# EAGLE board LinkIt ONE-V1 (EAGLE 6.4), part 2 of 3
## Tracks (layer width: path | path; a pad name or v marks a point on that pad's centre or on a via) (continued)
GND  (via drill 0.1 pad 0.25 layers 1-2, 0.1 pad 0.25 layers 15-16, 0.2 pad 0.41 (continued)
  Bottom 0.102: U7.F4 U7.D4 | U7.F6 U7.F7 | U7.F7 U7.G7 | U7.H6 U7.H7 U7.H8 U7.J8 | U7.H6 U7.G6 U7.F6 | U7.J6 U7.J5 | U7.J6 U7.H6 | U7.J6 U7.K6 | U7.J6 U7.J7 | U7.J7 35.34,76.69 35.38,76.73 U7.J8 | U7.J7 35.38,76.33 | U7.F6 36.6,75.93 36.6,75.92 36.55,75.92 | U7.N8 U7.N9 | U7.E2 36.94,74.58 v36.96,74.6 | U3.PAD 36.2,83.34 36.2,82.98 37.47,81.71 37.47,81 36.96,80.49 v36.7,80.49 36.5,80.49 36.14,80.85 34.98,80.85 | 34.98,80.85 v31.42,80.85 | 62.89,97.59 X2.2 62.98,97.36 | X2.1 62.98,97.36 | U7.L2 U7.L1 | 32.73,73.73 32.87,73.87 33.33,74.33 U7.P2 v33.35,74.35 | 62.98,97.36 C38.2 | C38.2 | v34.98,80.8 34.98,80.85 | U7.G2 36.16,74.33 36.45,74.04 36.45,73.25 35.38,72.19 v35.38,72.06 | U7.F7 v36.55,76.33 | C131.2 C129.2 | U7.K1 | v43.16,79.53 43.21,79.58 43.16,79.63 | 43.54,80.01 43.69,80.01
  Bottom 0.127: 34.55,74.33 34.87,74.65 34.87,75.06 v35.33,75.51 | v31.85,75.21 32.74,75.21 33,75.46 33,76.07 | v36.6,72.06 36.6,72.62 37.01,73.03 37.01,73.63
  Bottom 0.132: v38.05,69.29 38.94,68.4 | v41.68,75.97 41.45,75.97 arc45 41.11,75.83 41.02,75.74 arc-45 40.72,75.62 39.52,75.62
  Bottom 0.152: U2.14 56.54,93.32 56.71,93.15 59.56,93.15 C37.2 | 53.74,82.07 U1.E1 53.51,82.3 52.02,82.3 v51.89,82.42 | U1.K1 53.76,85.16 v53.37,85.55 | v43.21,75.21 43.16,75.21 43.05,75.31 | 43.05,75.31 41.52,75.31 arc45 41.27,75.21 41.02,74.95 v41.02,74.85 | U2.29 54.14,96.17 54.65,96.69 U2.PAD | 43.05,75.31 45.47,75.31 47.45,73.33 50.22,73.33 | U7.D4 U7.C5 U7.B6 | v40.56,70.08 40.56,69.93 40.97,69.52 47.37,69.52 50.27,72.41 v51.33,72.41 | v38,72.72 38,70.46 41.04,67.41 arc45 41.48,67.23 48.29,67.23 49.25,68.2 52.65,68.2 | 51.03,73.33 v51.33,73.33 v52.86,73.33 v54.28,73.33 v55.8,73.33 | v6.43,94.36 6.43,95.07 J4.C5 | v16.51,88.9 16.51,87.83 15.39,86.71 15.39,74.76 19.04,71.1 27.92,71.1 29.9,73.08 | 25.42,72.62 26.29,71.75 27.63,71.75 29.62,73.74 32.74,73.74 32.87,73.87 | 31.57,72.52 31.32,72.77 30.43,72.77 28.65,70.99 28.65,70.41 28.57,70.33 | v55.12,64.03 55.09,64.01 55.09,62.61 54.74,62.25 54.62,62.25 R56.2 53.98,61.59 53.21,61.59 52.07,62.74 52.07,63.22 v52.17,63.32 52.15,63.32 52.2,63.27 52.86,63.27 53.54,63.96 C130.2 | 28.88,76.48 28.88,76.38 29.39,75.87 30.45,75.87 30.99,75.34 v31.47,75.34 | 53.98,78.26 53.98,79.02 54.38,79.43 54.53,79.43 54.74,79.63 | X3.4 44.55,74.62 v44.81,74.88 | 43.16,79.63 43.54,80.01 | 43.16,79.58 v43.16,79.53 v43.16,78.97 42.69,78.5 C113.2 | 45.29,79.98 v45.29,80.03 | 50.93,64.4 R75.1 | v40.46,69.11 40.46,68.78 41.15,68.1 v41.38,68.1 | v38.68,72.72 38.68,70.79 39.5,69.98 | v39.29,72.67 39.29,71.45 39.75,70.99 | v37.36,72.47 v37.36,71.4 | v37.36,71.4 37.34,71.37 | v37.36,71.4 37.36,71.37 37.39,71.35 37.39,70.03 37.44,69.98 | 58.55,81.3 58.8,81.3 59.46,80.64 v60.12,80.64
  Bottom 0.152: R6.2 49.82,82.21 | U7.M3 U7.L2 34.55,74.33 | v35.38,72.06 35.38,70.74 34.93,70.28 34.87,70.28 34.72,70.13
  Bottom 0.203: 45.8,77.44 C110.2 45.61,77.48 45.29,77.8 45.29,79.98 45.03,80.24 L15.1 | 59.13,75.26 69.84,75.26 v70.07,75.49 | v72.16,77.34 72.19,77.32 72.19,75.97 70.62,74.41 47.67,74.41 46.1,75.97 v45.54,75.97 v44.73,75.97 | U2.8 55.16,96.17 54.65,96.69 | U2.46 56.14,98.56 55.63,98.04 | 55.26,82.1 U1.F4 U1.F6 U1.F7 | 15.47,97.81 JTAG.2 | v44.73,75.97 44.7,75.95 | v44.73,75.97 44.09,75.97 | 44.09,75.97 44.07,75.95 | 44.09,75.97 v43.21,75.97 | v43.21,75.97 43.18,75.95 | v43.21,75.97 42.44,75.97 | 42.44,75.97 42.42,75.95 | 42.44,75.97 v41.68,75.97 41.66,75.95 | U7.J5 v35.33,75.53 | v35.33,75.53 U7.J8 U7.H8 | U7.H8 | U7.H8 U7.H6 | 46.1,77.24 48.03,75.31 54.72,75.31 C15.2 | v35.33,75.53 v35.33,75.52 v35.33,75.51 | U1.E1 53.76,82.13 53.57,82.32 51.99,82.32 v51.89,82.42 | U1.D4 55.26,82.1 | 55.26,82.1 v55.27,82.12 | 58.95,72.41 58.95,72.31 | 58.95,71.65 v58.95,71.6 | U1.C5 56.13,80.67 v56.66,80.67 | U1.B8 57.26,80.92 v57.23,80.95 | U1.D9 57.29,81.55 v57.28,81.56 | 58.6,84.4 58.6,84.45 58.6,84.58 v59.05,85.04 | 50.85,80.55 v50.81,80.58 | v10.52,59.89 10.59,59.89 10.74,59.74 12.75,59.74 12.93,59.92 12.93,61.82 12.95,61.85
  Bottom 0.254: 40.72,76.33 v40.74,76.3 40.16,76.3 v39.8,76.66 | 36.54,75.77 U7.F6 U7.H6 34.93,75.93 34.93,75.92 | 36.54,75.77 36.54,75.14 36.55,75.13 U7.D4 | 35.38,76.33 U7.H7 | U7.G7 U7.H7 | U7.G7 v36.55,76.33 36.55,75.77 36.54,75.77 | U7.G7 U7.G6 | U7.H7 U7.H6 | U7.H7 U7.H8 | U7.D4 U7.D2 U7.E2 36.96,74.33 v36.96,74.6 | U7.A2 38.65,74.33 v38.99,73.99 | 39.73,76.73 v39.8,76.66 | U7.A8 38.68,76.73 38.79,76.83 39.62,76.83 v39.8,76.66 | v58.61,79.9 58.41,79.9 U1.A10 U1.B9 57.73,80.55 | 57.75,81.53 U1.D9 U1.D7 U1.D6 U1.C6 56.26,81.03 | U1.B1 53.42,80.55 53.32,80.44 50.95,80.44 v50.81,80.58 | U7.L2 v34.54,73.94 v34.56,73.93 U7.K1
  Bottom 0.305: J4.P5 18.79,92.42 18.67,92.3 18.67,87.07 17.68,86.08 17.68,81.24 18.66,80.26 20.83,80.26 23.97,77.12 28.24,77.12 28.88,76.48 28.9,76.45 C76.2 | C60.2 25.42,72.62 24.81,72.01 19.13,72.01 16.38,74.76 16.38,86.61 17.6,87.83 17.6,89.43 17.3,89.74 16.64,89.74 | C38.2 60.08,97.19 60.33,96.95 60.33,96.3 C39.2 | 16.64,89.74 15.72,89.74 15.37,89.38 15.37,87.81 14.4,86.84 14.4,74.78 18.85,70.33 28.57,70.33 28.8,70.33 30.37,68.77 34.38,68.77 34.72,69.11 34.72,70.02 C92.2 | 16.64,89.74 v16.66,89.76 | 57.73,80.55 57.73,80.54 | U1.C9 U1.B9 | U1.B8 | v77.52,99.95 77.57,99.9 GPS.GND1 80.85,99.9 81.61,100.66 GPS.GND3 81.61,101.93 80.85,102.69 GPS.GND2 78.31,102.69 v78.18,102.56 | WI-FI/BT.GND1 83.9,81.91 84.2,82.22 WI-FI/BT.GND3 84.2,84 83.49,84.71 WI-FI/BT.GND2 80.92,84.71 v80.8,84.58 | WI-FI/BT.GND1 82.57,81.91 82.52,81.97 | 82.52,81.97 82.63,81.97 WI-FI/BT.GND1 | 82.52,81.97 80.87,81.97 v80.8,82.04 | v80.77,66.8 80.9,66.93 GSM.GND2 83.59,66.93 84.2,66.32 GSM.GND3 84.2,64.8 83.54,64.13 GSM.GND1 80.9,64.13 v80.64,64.39 | v55.75,74.35 57.07,74.35 57.12,74.3 | X3.2 41.94,72.59 v42.24,72.29 | v50.81,80.58 50.41,80.58 49.86,80.03 49.86,79.9 C6.2
  Bottom 0.406: C26.2 C39.2 | C38.2 60.08,97.88 v60.07,97.89 | C42.2 55.55,102.79 | C5.2 v33.02,95.4 33.05,95.38 | 53.98,78.26 53.98,77.65 53.57,77.24 v53.57,76.28 | C66.2 23.47,86.61 25.02,85.06 | C6.2 49.4,79.86 v49.39,79.87 | U11.35 65.02,81.41 | U11.35 66.17,80.14 | U11.35 66.17,82.55 | 67.31,81.41 U11.35 | v13.18,76.53 13.18,74.45 18.54,69.09 28.47,69.09 29.8,67.76 35.12,67.76 36.07,68.71 36.07,69.96 R104.2
  Bottom 0.457: 50.22,73.33 50.76,73.33 | 55.83,73.33 51.03,73.33 47.07,73.33 46.86,73.53
  Bottom 0.508: 55.83,73.33 56.01,73.15 58.12,73.15 58.95,72.31 58.95,71.65
  other vias: 34.14,77.93 36.54,75.13 36.54,75.53 35.34,76.33 35.73,75.93 35.74,76.56 33.74,77.13 38.68,71.86 37.41,69.98 38.73,70.82 39.5,73.48 40.16,71.96 40.92,71.3 40.51,73.89 42.34,71.63 41.02,73.89 40.67,75.59 42.39,75.97 44.02,75.97 45.49,75.16 42.8,75.16 43.61,75.16 44.37,75.16 45.14,75.16 45.14,76.17 44.37,76.17 43.61,76.23 42.8,76.23 31.17,81.76 41.22,76.83 58.29,101.73 61.09,101.73 61.98,101.73 61.09,99.82 61.98,99.82 59.82,99.82 62.99,99.82 62.99,103 64.26,103 65.53,103 66.8,103 68.07,103 68.96,98.81 68.96,99.82 68.07,100.97 69.34,103 70.61,103 71.88,103 73.15,103 70.61,100.46 71.88,100.46 73.15,100.46 75.06,103 75.06,100.46 76.17,100.46 52.93,88.44 78.13,84.58 78.13,83.31 78.26,82.04 79.53,82.04 78.26,80.77 79.65,81.15 77.9,77.72 75.59,77.6 75.46,79.88 79.4,79.12 59.99,78.41 60.63,77.65 61.43,77.09 62.76,76.96 64.16,76.96 65.11,76.96 65.18,79.38 63.59,79.38 62.32,79.38 61.37,79.18 60.76,80.09 67.74,76.81 70.05,79.76 68.35,79.76 71.2,79.76 72.39,79.76 72.92,76.96 70.03,76.23 51.31,75.31 57.84,75.34 45.29,77.9 45.29,78.97 44.53,80.9 44.58,70.84 42.34,70.94 52.86,72.42 54.28,72.42 55.17,72.42 51.33,71.5 52.86,71.5 54.28,71.5 51.36,69.52 52.71,69.32 51.89,66.88 78.84,78.1 61.37,73.91 42.6,62.76 45.21,64.97 46.28,64.97 47.29,64.97 49.28,62.94 39.93,67.36 39.52,69.95 39.29,67.89 40.41,67.03 59.82,68.07 61.72,68.07 61.72,69.98 62.99,69.98 64.26,69.98 65.53,69.98 66.8,69.98 68.07,69.34 66.8,68.07 65.53,68.07 64.26,68.07 62.99,68.07 70.48,64.9 69.6,67.94 68.07,66.8 71.25,66.55 69.34,65.53 73.02,66.29 71.88,64.9 74.55,66.17 75.69,66.8 75.56,64.9 73.79,64.9 77.6,66.8 77.6,64.9 79.38,64.9 26.59,77.7 24.71,80.54 25.78,79.43 22.58,80.7 23.9,81.36 20.9,82.17 14.35,83.77 14.4,81.86 16.38,81.81 16.38,83.77 17.65,81.81 7.65,81.2 9.22,81.15 10.54,81.15 16.46,77.72 25.25,103 21.74,102.21 54.74,96.65 55.73,89.18 56.03,90.09 59.69,89.13 55.55,103 54.28,102.97 56.92,103 50.62,102.69 52.83,98.55 54.74,98.55 56.64,98.55 52.83,96.65 56.64,96.65 56.64,94.74 54.74,94.74 52.83,94.74 55.42,85.5 19.66,94.18 19.71,92.91 13.72,97.08 6.81,98.7 28.37,94.87 29.34,92.63 11.1,83.03 24.61,75.26 24.66,74.55 24.66,73.74 36.6,75.21 38.89,73.63 38.89,73.08 33.81,74.09 38.13,82.42 38.58,82.42 36.75,82.47 35.59,82.47 34.26,82.47 50.04,62.92 42.34,68.22 40.21,72.92 40.82,72.31 12.6,91.85 20.75,80.34 18.62,80.29 17.3,79.76 54.64,69.95 56.03,69.95 57.56,69.95 56.03,68.68 57.56,68.68 54.64,68.68 54.64,67.41 55.91,67.41 57.56,67.41 53.85,98.55 55.75,98.55 53.72,96.65 55.75,96.65 53.72,94.74 55.75,94.74 52.83,95.63 52.83,97.66 53.85,97.66 54.74,97.66 55.75,97.66 56.64,97.66 56.64,95.63 55.75,95.63 54.74,95.63 53.72,95.63 44.45,74.63 44.02,75.26 44.73,75.26 42.42,75.26 41.66,75.29 39.27,71.86 39.55,71.15 40.01,70.69 36.96,69.42 37.47,69.42 38.96,69.44 38,71.86 38,70.84 38.38,70.03 39.85,68.55 52.55,68.2 52.1,71.5 57.84,74.32 51.33,74.3 52.86,74.3 54.23,74.35 52.86,75.31 57.12,73.15 36.52,75.92 37.01,74.88 37.36,74.42 37.8,73.99 31.17,82.83 31.17,84 30.86,80.24 29.95,80.99 29.79,84.25 40.69,78.33 33.12,74.04 15.37,83.77 15.37,81.86 15.37,80.31 16.38,80.31 14.4,80.31 29.84,73.08 21.03,92.86 21.69,93.22 22,94.34 20.57,93.62 49.05,95.2 49,96.22 44.58,69.52 44.58,68.38 46.46,71.81 46.46,70.84 46.46,69.52 46.41,68.38 27.41,77.72 27.18,80.44 25.2,80.01 44.58,66.47 37.29,73.43 37.85,73.43 38.46,73.43 38.46,73.99 13.18,80.37 13.18,77.7 17.4,77.7 36.65,72.62 35.43,71.45 2.03,92.89 2.03,90.35 5.33,92.89 5.21,90.22 2.03,87.81 5.21,87.81 15.37,58.55 16.64,58.55 58.04,62.79 60.45,62.36 62.99,62.36 62.99,64.26 62.99,66.17 59.82,66.17 70.61,61.72 73.79,61.72 75.82,61.72 78.23,61.72 81.41,57.28 81.41,61.72 61.72,70.99 65.91,73.91 70.61,57.28 70.1,73.91 69.34,70.61 76.96,73.91 76.96,70.36 82.04,73.79 82.04,70.61 69.98,84.58 75.95,82.04 69.98,92.2 75.69,92.2 82.04,92.2 68.96,97.92 80.14,97.92 55.37,88.39 57.28,88.39 0.89,78.1 50.72,85.6 12.19,98.6 12.19,101.14 10.29,101.14 5.21,101.14 10.29,107.37 28.52,73.36 71.88,78.36 66.67,78.1 30.58,75.21 30.58,73.94 32.77,71.81 32.61,73.66 32.61,73.03 31.8,73.08 35,72.69 35.56,72.69 48.64,91.08 24.99,85.09 22.35,90.32 31.22,77.11 41.96,78.45 41.2,78.33 41.2,77.88 40.69,77.88 35.71,78.08 34.7,78.03 36.88,76.17 36.6,75.82 40.94,67.46 48.69,75.82 48.74,72.44 48.74,69.01 48.74,69.65 25.29,73.72 42.47,66.45 30.61,73.48 31.32,73.48 30.61,72.57 31.32,72.57 30.58,73.05 31.45,74.04 62.76,73.91 64.03,73.91 58.7,75.31 58.7,74.3 68.22,73.91 23.13,79.77 36.17,72.69 32.74,72.42 42.82,80.21 61.77,87.76 32.49,103.38 38.84,103.25 42.52,100.33 43.03,96.52 46.71,102.74 46.71,100.46 46.71,98.04 49,93.47 50.77,90.55 51.41,91.19 38.33,90.3 19.81,58.55 19.81,57.91 77.01,77.72 77.01,78.99 78.03,79.5 75.49,78.87 75.95,83.31 76.07,85.85 33.07,71.02 34.29,71.02 35.51,71.02 31.8,71.02 59.11,79.43 48.4,76.52 59.82,73.91 59.82,71.88 61.72,71.88 70.03,77.5 59.66,85.55 64.48,79.38 30.2,61.54 33.76,61.67 32.11,61.54 35.92,67.13 36.68,67.13 37.44,67.13 39.09,67.39 39.47,66.75 20.04,67.26 20.68,67.26 21.31,67.26 15.19,67.34 10.52,68.4 13.94,62.56 13.18,62.81 13.44,67.39 18.67,72.87 19.18,72.36 22.35,75.41 22.35,74.27 21.84,74.78 30.58,69.42 35.69,75.62 34.01,75.72 34.95,73.94 34.19,73.61 73.79,57.28 75.69,57.28 78.23,57.28 19.3,73 22.22,58.04
  pour GND1 (isolate 0.152, no thermals): 35.18,76.71 36.7,76.71 36.7,75.69 35.18,75.69
  pour GND (isolate 0.254, no thermals): 38.33,74.6 41.43,74.6 41.43,76.58 38.33,76.58
  pour Top (isolate 0.254, rank 4): -0.13,109.98 73.91,109.85 73.79,98.55 73.79,55.24 -0.89,55.37 -0.89,109.98
  pour Bottom (isolate 0.254, rank 3): -0.13,109.98 73.91,109.85 73.66,55.24 -0.89,55.37 -0.89,109.98
  pour Top (isolate 0.254, rank 6, no thermals): 3.3,56.01 39.5,56.01 39.5,59.82 44.58,59.82 44.58,56.01 85.22,56.01 85.22,62.99 81.41,62.99 81.41,68.07 85.22,68.07 85.22,80.77 81.41,80.77 81.41,85.85 85.22,85.85 85.22,98.55 78.87,98.55 78.87,103.63 84.58,103.63 84.58,109.35 28.07,109.35 28.07,105.54 24.89,105.54 24.89,109.35 0.13,109.35 0.13,95.38 5.21,95.38 5.21,76.33 0.13,76.33 0.13,67.44 10.29,67.56 10.29,61.72 3.3,61.72
  pour Bottom (isolate 0.254, rank 6, no thermals): 0.13,56.01 39.5,56.01 39.5,59.82 44.58,59.82 44.58,56.01 85.22,56.01 85.22,62.99 81.41,62.99 81.41,68.07 85.22,68.07 85.22,80.77 81.41,80.77 81.41,85.85 85.22,85.85 85.22,98.55 78.87,98.55 78.87,103.63 84.58,103.63 84.58,109.35 28.07,109.35 28.07,105.54 24.89,105.54 24.89,109.35 0.13,109.35 0.13,95.38 5.21,95.38 5.21,76.33 0.13,76.33 0.13,67.44 10.29,67.56 10.29,65.02 0.13,64.9
  pour GND (isolate 0.254, rank 6): -0.51,56.01 85.22,56.01 85.22,62.99 81.41,62.99 81.41,68.07 85.22,68.07 85.22,80.77 81.41,80.77 81.41,85.85 85.22,85.85 85.22,98.55 78.87,98.55 78.87,103.63 84.58,103.63 84.58,109.35 -0.51,109.35
  pour GND1 (isolate 0.254, rank 6): -1.14,56.01 85.22,56.01 85.22,62.99 81.41,62.99 81.41,68.07 85.22,68.07 85.22,80.77 81.41,80.77 81.41,85.85 85.22,85.85 85.22,98.55 78.87,98.55 78.87,103.63 84.58,103.63 84.58,109.35 -1.14,109.35
GNSS_CORE_1V1  (via drill 0.3 pad 0.51)
  Top 0.406: 55.25,100.08 53.31,100.08 51.82,98.59 51.82,94.36 v51.18,93.73 | 55.25,100.08 56.64,100.08 58.42,98.3 v58.42,96.95 58.42,95.12 58.04,94.74 v58.04,93.73 | v55.3,100.69 55.3,100.13 55.25,100.08
  Bottom 0.152: U2.43 54.94,100.33 v55.3,100.69 55.51,100.9 55.51,101.03
  Bottom 0.203: 56.94,93.58 U2.13 56.98,93.73 v58.04,93.73 59.25,93.73 C37.1 | C42.1 55.51,101.03 | 55.63,101.09 55.5,101.09 55.5,100.89 v55.3,100.69 | U2.24 51.23,93.77 v51.18,93.73 50.27,93.73 C41.1 | U2.6 58.4,96.97 v58.42,96.95
  Bottom 0.406: C41.1 50.11,94.06
GNSS_DCV
  Bottom 0.203: 59.56,91.82 59.69,91.82 L3.1
  Bottom 0.254: U2.15 56.14,93.07 56.49,92.71 56.64,92.71
  Bottom 0.305: 59.56,91.82 58.67,92.71 57.15,92.71 56.64,92.71 56.49,92.71 56.26,92.94
GNSS_DCV_1V8  (via drill 0.3 pad 0.51)
  Top 0.406: 55.34,93.45 C44.1 55.21,93.32 v55.21,92.63
  GND 0.406: 57.53,99.44 57.53,99.8 56.11,101.22 56.04,101.29 52.27,101.29 v52.2,101.22 | v60.83,90.17 58.29,90.17 57.28,91.19 57.28,92.46 | v58.29,99.31 57.66,99.31 57.53,99.44 | 57.53,99.44 57.53,94.34 v57.46,94.26 57.28,94.08 57.28,92.84 | 57.28,92.46 57.28,92.84 | v55.21,92.63 57.07,92.63 | 57.07,92.63 57.28,92.84 | 57.07,92.63 57.1,92.63 57.28,92.46
  Bottom 0.152: v57.46,94.26 57.46,94.49 57.53,94.56 57.73,94.56 U2.12
  Bottom 0.203: U2.17 55.34,92.76 v55.21,92.63 | U2.4 58.21,97.77 58.42,97.99 58.42,98.81 58.25,98.97 | U2.1 58.25,98.97 | 58.25,98.97 58.25,99.27 v58.29,99.31
  Bottom 0.406: 59.41,90.09 L3.2 59.82,90.17 v60.83,90.17 | C34.1 51.51,101.22 v52.2,101.22 52.2,101.35 52.71,101.85 | 52.71,101.85 52.95,101.85 R80.1 52.77,101.92 52.71,101.85
GNSS_EN  (via drill 0.1 pad 0.25 layers 15-16, 0.2 pad 0.41 layers 2-15, 0.3 pad 0.51)
  Top 0.152: U4.3 54.36,89.2 54.36,88.47 53.79,87.9 52.54,87.9 51.61,88.82 47.83,88.82 46.81,89.84 41.99,89.84 40.97,88.82 38.49,88.82 38.02,89.29 37.85,89.47 37.85,90.78 v38.02,90.96
  GND 0.152: v39.01,82.5 38.89,82.63 38.89,90.45 38.38,90.96 v38.02,90.96
  GND1 0.076: v37.73,77.54 38.04,77.54 38.22,77.36 38.54,77.36 38.86,77.68 39.24,77.68 39.8,78.24 39.8,78.72 39.45,79.07 39.45,80.11 39.57,80.24 39.57,81.94 v39.01,82.5
  Bottom 0.076: 37.34,76.76 U7.D8 37.33,76.93 37.73,77.32 v37.73,77.54
GNSS_FRAME_SYNC  (via drill 0.3 pad 0.51)
  Top 0.152: v48.9,98.37 48.49,97.97 48.49,91.77 47.88,91.16 | 47.88,91.16 47.68,90.96 v47.68,89.64 | 47.88,91.16 41.48,91.16 41.2,90.88 v41.2,90.81
  GND 0.152: v47.68,89.64 47.68,86.28 47.32,85.93 47.32,83.87 45.97,82.53 44.93,82.53 v44.78,82.37 | v21.49,99.62 22.05,99.62 22.48,99.19 31.57,99.19 32.79,97.97 34.47,97.97 38.02,94.41 38.36,94.41 41.2,91.57 v41.2,90.81
  Bottom 0.076: U7.B12 37.9,78.58 37.9,78.91 37.99,79 38.11,79 38.15,79.05
  Bottom 0.102: 42.6,80.9 42.6,80.75 42.6,80.5 41.87,79.78 38.89,79.78 38.15,79.05
  Bottom 0.152: 42.6,80.75 42.6,82.12 43.26,82.78 44.37,82.78 v44.78,82.37 | v48.9,98.37 R26.1 | v21.49,99.62 21.21,99.34 21.21,98.02 21.51,97.71 21.51,96.42 21.26,96.17 20.81,96.17 20.55,96.43 20.55,96.65 19.98,97.22 R65.1
GNSS_HRST  (via drill 0.1 pad 0.25 layers 15-16, 0.2 pad 0.41 layers 2-15, 0.3 pad 0.51)
  Top 0.152: v57.53,101.85 56.9,102.49 51.59,102.49 50.67,101.57 50.67,100.93 50.35,100.61 48.1,100.61 47.57,100.09 47.57,92.23 47.47,92.13 37.3,92.13 35.18,90.01 v35.18,89.74
  GND 0.152: v36.2,81.3 36.2,81.41 36.3,81.51 36.3,85.98 34.37,87.91 34.37,88.92 v35.18,89.74
  GND1 0.152: v36.2,81.3 36.2,80.64 v36.04,80.49
  Bottom 0.076: U7.H12 35.5,78.57 35.5,79.26 35.74,79.5 35.74,80.19 v36.04,80.49
  Bottom 0.152: R52.1 57.47,101.92 v57.53,101.85
GNSS_REF
  Bottom 0.152: U2.7 58.11,96.57 58.29,96.39 58.67,96.39 59.18,96.9 59.18,97.35 C38.1
GNSS_TXIND  (via drill 0.1 pad 0.25 layers 15-16, 0.2 pad 0.41 layers 2-15, 0.3 pad 0.51)
  GND 0.152: v41.49,79.62 41.49,79.89 42.6,81 42.6,84.76 44.88,87.05 44.88,87.53 47.9,90.55 49.91,90.55 51.79,92.43 51.79,93.8 v51.05,94.54
  GND1 0.076: 36.96,75.89 36.98,75.89 U7.E6 37.05,75.82 40.08,75.82 40.36,76.1 40.36,76.35 40.46,76.45
  GND1 0.102: U7.E6 36.95,75.93 | 40.92,76.91 | 40.92,76.91 40.92,77.04 41.33,77.44 41.33,79.46 v41.49,79.62 | 40.92,76.91 40.46,76.45
  Bottom 0.152: U2.25 51.09,94.57 v51.05,94.54
  other vias: 36.94,75.93
GNSS_UART_RX  (via drill 0.1 pad 0.25 layers 15-16, 0.2 pad 0.41 layers 2-15, 0.3 pad 0.51)
  Top 0.152: v48.95,99.19 48.18,98.42 48.18,91.92 47.73,91.47 37.52,91.47 36.6,90.55 v36.6,89.74
  GND 0.152: 36.6,89.89 v36.6,89.74 38,88.34 38,81.94 38.1,81.84 v38.12,81.84
  GND1 0.102: v38.23,80.44 38.23,81.66 38.23,81.71 38.23,81.74 v38.12,81.84
  Bottom 0.102: U7.E13 36.94,79.26 38.12,80.44 v38.23,80.44
  Bottom 0.152: U2.35 51.16,98.57 50.55,99.19 v48.95,99.19
GNSS_UART_TX  (via drill 0.1 pad 0.25 layers 15-16, 0.2 pad 0.41 layers 2-15, 0.3 pad 0.51)
  Top 0.152: v35.89,89.74 35.89,90.28 37.38,91.77 47.57,91.77 47.88,92.07 47.88,99.14 v48.54,99.8
  GND 0.152: v35.89,89.74 37.72,87.91 37.72,81.48 v37.85,81.36 | v21.06,96.65 21.06,96.85 22.17,97.97 27.15,97.97 29.08,96.04 33.85,96.04 36.4,93.49 36.4,90.45 35.89,89.94 v35.89,89.74 | v35.89,89.74 35.89,89.79
  GND1 0.076: U7.D10 37.07,77.8 37.07,78.07 37.72,78.72 37.72,81.23 v37.85,81.36
  Bottom 0.152: v21.06,96.65 21.21,96.8 21.21,97.56 20.9,97.87 20.9,99.96 R63.1
  Bottom 0.203: U2.37 48.56,99.77 v48.54,99.8
  other vias: 37.34,77.53
GNSS_VGNSS_MAIN  (via drill 0.3 pad 0.51)
  Top 0.406: C46.1 58.42,91.19 v58.42,91.87 58.47,91.87 59.82,93.22 59.82,96.52 v59.64,96.7
  Top 0.61: U4.5 58.49,91.12 C46.1
  Bottom 0.203: 56.72,92.13 57.12,92.13 57.23,92.02 C35.1 | U2.16 55.74,92.28 C31.2 | U2.9 58.91,95.77 C39.1
  Bottom 0.406: C31.2 57.09,92.16 57.23,92.02 | C39.1 59.2,96.25 v59.64,96.7
  Bottom 0.61: v58.42,91.87 C35.1
GNSS_VRTC_1V1
  Bottom 0.203: U2.18 54.94,93.16 54.36,92.58 54.36,91.85 54.37,91.83
  Bottom 0.406: C31.1 54.93,91.28 54.37,91.83 C99.1
GNSS_VRTC_4V3  (via drill 0.3 pad 0.51)
  Top 0.406: R7.1 14.83,86.49 D1.- | D1.- 14.91,86.59 | v51.08,87.43 47.42,87.43 46.43,88.42 42.39,88.42 41.46,87.48 37.64,87.48 37.01,88.11 35.89,88.11 35.33,87.55 34.78,87.55 33.5,88.82 v33.5,88.88 | D1.- 14.48,87.05 14.45,87.05 14.45,87.15 14.4,87.15 v14.12,87.43
  GND 0.406: v14.12,87.43 14.21,87.34 18.71,87.34 19.28,87.91 19.28,89.94 21.01,91.67 v21.01,91.69
  Bottom 0.203: U2.19 54.54,93.32 53.95,92.73 53.51,92.73 C29.1
  Bottom 0.406: C29.1 52.46,92.22 52.2,91.95 52.2,88.54 v51.08,87.43 | v33.5,88.88 32.84,88.21 27.71,88.21 24.23,91.69 v21.01,91.69
GNSS_VTCXO_SW  (via drill 0.3 pad 0.51)
  GND 0.254: v60.45,94.36 60.91,93.91 66.8,93.91 | 66.8,93.91 69.78,93.91 70.1,94.23 v70.1,95.88 | 67.03,94.13 67.03,95.82 v67.02,95.83 | 67.03,94.13 66.8,93.91 | 67.03,94.13 67.25,93.92
  Bottom 0.152: C26.1 59.2,95.36 | 64.26,95.78 X2.4 66.98,95.8 v67.02,95.83 66.99,95.86 C120.1 66.97,99.33 C119.1 66.95,100.2 R41.2 65.91,100.27 65.91,100.58 65.66,100.84 64.01,100.84 64.05,100.79 U13.4 | C26.1 59.74,94.63 60.44,94.63 60.45,94.61 v60.45,94.36 | U2.10 58.99,95.37 C26.1
  Bottom 0.254: v70.1,95.88 70.1,98.04 C80.1 70.17,99.44 L20.2
GNSS_VTLDO  (via drill 0.3 pad 0.51)
  Top 0.406: C36.1 58.75,94.39 v58.85,94.49 59.05,94.7 59.05,99.44 56.57,101.93 v54.66,101.93 51.77,101.93 51.18,101.35 51.18,100.76 49.76,99.34 49.76,97.77 | 49.76,97.77 49.76,97.16 | 49.76,97.16 49.76,95 v49.73,94.97 | v48.95,97.48 R31.1 | R31.1 49.48,97.48 49.76,97.77 | R31.1 49.76,97.16
  Bottom 0.152: U2.11 58.36,94.97 v58.85,94.49 | U2.42 54.54,100.51 54.74,100.71 54.74,101.85 v54.66,101.93
  Bottom 0.203: U2.30 51.11,96.57 50.88,96.34 50.88,95.91 50.7,95.73 50.36,95.73 C40.1 50.36,95.68 50.37,95.68 | R31.1 v48.95,97.48
  Bottom 0.406: 50.37,95.69 50.37,95.68 50.37,95.32 50.04,95 49.76,95 v49.73,94.97
GPIO0/ADC0/U3RX  (via drill 0.1 pad 0.25 layers 1-2, 0.1 pad 0.25 layers 15-16, 0.2 pad 0.41 layers 2-15, 0.3 pad 0.51)
  Top 0.152: R59.1 45.02,63.39 | R59.1 44.54,63.99 v44.54,64.9 | v44.54,64.9 44.54,65.01 | R88.1 R59.1 | v44.54,64.9 44.54,65.11 45.06,65.63 45.06,72.95 43.61,74.4 v43.61,78.82
  GND 0.152: v36.73,77.12 | v36.73,77.12 39.01,77.12 v39.1,77.21 | v40.01,79.27 41.17,79.27 41.53,78.92 43.51,78.92 v43.61,78.82
  GND1 0.076: U7.F8 36.54,76.81 36.73,77 v36.73,77.11 v36.73,77.12 | v39.1,77.21 39.31,77.21 40.16,78.06 40.16,79.12 v40.01,79.27
  Bottom 0.152: 46.66,64.49 48.04,64.49 C103.1 | 46.66,64.49 46.51,64.49 | 46.51,64.49 44.94,64.49 v44.54,64.9 | U17.4 46.59,64.41 | 46.59,64.41 46.59,64.42 46.66,64.49 | 46.59,64.41 46.51,64.49
  other vias: 36.54,76.73
GPIO1/ADC1/U3TX  (via drill 0.1 pad 0.25 layers 1-2, 0.1 pad 0.25 layers 15-16, 0.2 pad 0.41 layers 2-15, 0.3 pad 0.51)
  Top 0.152: R89.1 46.25,62.97 | 46.25,62.97 C102.1 46.09,63.39 45.7,63.78 45.7,65.3 45.34,65.66 45.34,73.08 43.97,74.44 43.97,79.73 v44.37,80.14 | v45.9,62.97 46.25,62.97
  GND 0.152: v43.36,80.39 44.12,80.39 v44.37,80.14
  GND1 0.102: v42.29,80.59 43.16,80.59 v43.36,80.39
  Bottom 0.076: 36.96,79.58 36.69,79.31 36.69,78.56 36.92,78.33 U7.E12
  Bottom 0.102: 36.96,79.58 38.12,80.75 38.68,80.75 39.45,79.98 41.68,79.98 v42.29,80.59
  Bottom 0.152: v45.9,62.97 46.08,63.14 U17.5 46.89,63.14 47.37,63.63 R58.1
GPIO2/ADC2/PWM0  (via drill 0.1 pad 0.25 layers 15-16, 0.3 pad 0.51)
  Top 0.152: C89.1 47.23,63.36 | 47.23,63.36 46.81,63.78 46.81,65.11 45.62,66.29 45.62,73.2 44.27,74.55 44.27,79.55 45.57,80.85 v46,80.85 | R90.1 v47.37,62.86 47.37,63.22 47.23,63.36
  GND1 0.076: U7.D11 37.34,78.08 38.18,78.92 38.6,78.92 38.91,79.24 38.91,80.32 39.04,80.44 39.04,80.82 v38.94,80.92
  Bottom 0.152: v46,80.85 45.24,81.61 45.24,82.63 44.78,83.08 41.4,83.08 41.4,83.06 39.27,80.92 v38.94,80.92 | v47.37,62.86 R90.1 47.02,62 45.75,62 45.16,62.59 45.16,63.02 45.03,63.14 U17.2 43.99,63.14 43.71,62.86 43.71,62.55 R45.1
  other vias: 37.34,77.93
GPIO13/EINT11/PWM0  (via drill 0.1 pad 0.25 layers 15-16, 0.2 pad 0.41 layers 2-15, 0.3 pad 0.51)
  GND 0.152: 28.42,98.58 31.32,98.58 32.54,97.36 34.24,97.36 37.62,93.98 37.62,92.38 37.91,92.08 38.73,92.08 39.8,91.01 39.8,83.13 40.06,82.88 40.06,81.36 38.58,79.88 v38.43,79.88 | 28.42,98.58 21.11,98.58 20.19,97.66 20.19,96.05 20.56,95.68 v21.01,95.68 | 28.42,98.58 v28.42,98.37
  GND1 0.152: v38.17,79.75 38.3,79.75 v38.43,79.88
  Bottom 0.076: 37.35,78.33 U7.D12 37.35,78.33 37.58,78.56 37.58,79.34 37.99,79.75 v38.17,79.75
  Bottom 0.152: U18.4 29.57,96.71 28.42,97.87 v28.42,98.37 | R64.1 20.56,95.68 v21.01,95.68
GPIO19/PWM1  (via drill 0.1 pad 0.25 layers 15-16, 0.2 pad 0.41 layers 2-15, 0.3 pad 0.51)
  GND 0.152: v20.7,97.28 20.73,97.28 21.72,98.27 27.61,98.27 v27.76,98.12 27.76,97.81 29.03,96.55 29.03,96.54 29.23,96.34 33.98,96.34 36.7,93.62 36.7,90.45 38.28,88.88 38.28,82.27 38.61,81.94 v38.61,81.38
  GND1 0.076: U7.C11 37.74,78.23 38.28,78.77 38.77,78.77 39.09,79.09 39.09,80.24 39.27,80.41 39.27,80.98 38.86,81.38 v38.61,81.38
  Bottom 0.152: R66.1 20.02,98.3 20.7,97.61 v20.7,97.28 | U18.5 28.92,96.85 27.76,98.02 v27.76,98.12
  other vias: 37.74,77.93
GPIO40/SIM2_SIO  (via drill 0.1 pad 0.25 layers 15-16, 0.2 pad 0.41 layers 2-15, 0.3 pad 0.51)
  GND 0.152: v35.89,81.81 35.99,81.91 35.99,85.88 34.06,87.81 34.06,90.81 35.38,92.13 v35.84,92.13
  GND1 0.152: v35.64,80.49 35.64,80.59 35.79,80.75 35.79,81.71 v35.89,81.81
  Bottom 0.076: v35.64,80.49 35.56,80.42 35.56,79.59 35.34,79.38 U7.J12 35.34,78.35 35.33,78.36
  Bottom 0.152: Q10.2 36.51,94.47 R112.2 35.84,92.47 v35.84,92.13
GPIO_3/PWM1  (via drill 0.1 pad 0.25 layers 15-16, 0.2 pad 0.41 layers 2-15, 0.3 pad 0.51)
  GND 0.152: v38.63,80.59 38.88,80.59 39.75,81.47 39.75,82.73 39.5,82.98 39.5,90.75 38.48,91.77 37.77,91.77 37.31,92.23 37.31,93.86 34.22,96.95 32.23,96.95 v32.08,97.1
  GND1 0.152: v38.64,80.32 v38.64,80.59 v38.63,80.59
  Bottom 0.102: U7.D13 37.34,79.35 38.08,80.09 38.41,80.09 v38.64,80.32
  Bottom 0.152: U18.1 31.57,96.14 31.57,96.65 32.03,97.1 v32.08,97.1
GPS_RFIN
  Bottom 0.132: U2.48 56.94,99.99 57.42,100.47 arc-45 58,100.71 C67.2 59.25,101.6 L18.1
GPS_RTC_32K  (via drill 0.1 pad 0.25 layers 15-16, 0.2 pad 0.41 layers 2-15, 0.3 pad 0.51)
  GND 0.102: v35.27,79.08 36.75,77.6 39.29,77.6 39.8,78.1 39.8,78.72 39.45,79.07 39.45,79.63 39.7,79.88 40.73,79.88 40.79,79.93
  GND 0.152: 40.79,79.93 41.79,80.94 41.79,82.16 41.48,82.47 41.48,85.47 44.02,88.01 44.17,88.01 47.73,91.57 v49.15,91.57
  GND1 0.076: v35.27,79.08 35.34,79.01 v35.34,77.94 U7.J11
  Bottom 0.076: U7.J11 v35.34,77.94
  Bottom 0.152: U2.21 53.74,93.23 53.59,93.09 52.45,93.09 50.93,91.57 v49.15,91.57
ISENSE  (via drill 0.3 pad 0.51)
  GND 0.152: v33.27,70.1 33.05,70.33 29.52,70.33 28.65,71.2 13.49,71.2 11.2,73.48 5.61,73.48 4.65,72.52 v4.65,67.31
  Bottom 0.102: U7.H2 35.43,74.02 35.43,73.33 33.98,71.88 33.98,71.27 33.66,70.94 33.66,70.48 v33.27,70.1
  Bottom 0.406: 1.91,63.75 1.91,63.88 Q14.3
  Bottom 2.032: v4.65,67.31 2.79,67.31 1.91,66.42 1.91,64.13
  pour Bottom (isolate 0.254, no thermals): 2.79,62.33 2.79,64.52 arc90 2.54,64.77 1.27,64.77 arc90 1.02,64.52 1.02,59.05 arc90 1.27,58.8 3.43,58.8 3.43,62.08 3.05,62.08 arc-90
  pour Bottom (isolate 0.254, no thermals): 5.33,64.9 7.24,64.9 7.24,66.24 5.41,68.07 4.06,68.07 4.06,66.29 4.88,66.29 5.33,65.84
JTAG_2V8
  Bottom 0.203: JTAG.1 15.79,95.82 16.69,94.92 18.2,94.92 18.71,94.92 18.78,94.92 R38.2
JTCK
  Bottom 0.203: R65.2 18.18,97.28 JTAG.9
JTDI
  Bottom 0.152: R63.2 18.57,100.89 JTAG.7
JTDO
  Bottom 0.203: R66.2 19.09,98.37 JTAG.8
JTMS
  Bottom 0.203: R64.2 18.08,96.27 JTAG.10
JTRST_B
  Bottom 0.305: 17.65,103.81 JTAG.6 17.7,103.76 17.84,103.76 19.09,102.51 R39.2
JTRTCK
  Bottom 0.152: JTAG.4 15.64,101.61 16.54,100.71 18.25,100.71 R68.1
LPTE_MUX  (via drill 0.1 pad 0.25 layers 15-16, 0.2 pad 0.41 layers 2-15, 0.3 pad 0.51)
  Top 0.152: v32.23,95.53 32.64,95.94 34.6,95.94 34.77,95.94 39.4,95.94 v39.7,96.24
  GND 0.152: v34.14,78.79 34.14,79.3 33.1,80.34 32.39,80.34 32.03,80.7 32.03,89.71 33.94,91.62 33.94,93.72 32.23,95.43 v32.23,95.53
  GND1 0.076: v35.08,77.62 35,77.7 35,78.23 34.47,78.77 34.16,78.77 v34.14,78.79
  Bottom 0.076: U7.J10 35.17,77.53 v35.08,77.62
  Bottom 0.152: R118.2 40.2,94.09 Q13.2 39.7,94.59 v39.7,96.24
LSA0_LCM  (via drill 0.1 pad 0.25 layers 1-2, 0.1 pad 0.25 layers 15-16, 0.2 pad 0.41 layers 2-15)
  Top 0.254: R37.2 34.34,80.72 v34.67,80.39 35.45,80.39 R24.2
  GND 0.152: v35.37,76.81 35.37,78.02 35.34,78.04 34.82,78.56 34.82,79.38 34.47,79.73 34.47,80.19 v34.67,80.39
  GND1 0.076: U7.J9 35.34,76.84 v35.37,76.81
  other vias: 35.34,77.13
LSCE_B/EINT20  (via drill 0.1 pad 0.25 layers 15-16, 0.2 pad 0.41 layers 2-15, 0.3 pad 0.51)
  GND 0.152: v36.8,79.88 36.8,80.14 36.6,80.34 36.6,86.08 35.03,87.66 v35.03,88.16
  GND1 0.076: U7.G9 36.15,77.14 36.15,77.29 36.12,77.32 | 36.91,79.78 v36.8,79.88 36.8,79.5 35.94,78.64 35.94,77.73 36.03,77.63 36.03,77.4 36.11,77.32 36.12,77.32 | 36.12,77.32 36.11,77.33
  Bottom 0.152: v35.03,88.16 35.48,88.62 39.6,88.62 39.97,88.62 | 39.97,88.62 40.03,88.62 40.13,88.52 40.13,88.51 | Q11.2 39.88,89.66 39.88,89.53 40.2,89.22 R114.2 39.97,88.62
  other vias: 36.14,77.13
LSCK_LCM  (via drill 0.1 pad 0.25 layers 1-2, 0.1 pad 0.25 layers 15-16, 0.2 pad 0.41 layers 2-15)
  Top 0.152: 34.07,79.22 R97.1 34.02,79.27 v33.6,79.27
  GND 0.076: v33.6,79.27 33.6,79.08 33.61,79.07
  GND 0.152: v33.61,78.94 33.61,79.07 33.61,79.21 33.61,79.26 v33.6,79.27
  GND1 0.076: U7.L10 34.81,77.8 34.81,78.04 34.42,78.44 33.73,78.44 33.61,78.55 v33.61,78.94
  other vias: 34.54,77.53
LSDA_LCM/EINT21  (via drill 0.1 pad 0.25 layers 15-16, 0.2 pad 0.41 layers 2-15, 0.3 pad 0.51)
  GND 0.152: v33.15,78.56 33.2,78.51 33.76,78.51 33.91,78.36 34.32,78.36 34.57,78.61 34.57,79.22 33.15,80.64 32.64,80.64 32.33,80.95 32.33,89.59 34.56,91.81 34.62,91.87 34.72,91.97 v34.72,92.48
  GND1 0.076: U7.L11 34.21,78.26 33.45,78.26 v33.15,78.56
  Bottom 0.152: v34.72,92.48 35.13,92.48 35.69,93.04 35.69,95.22 35.94,95.48 37.75,95.48 39.96,97.69 40.58,97.69 40.87,97.97 40.87,98.42 | 40.87,98.42 40.87,98.68 | 40.87,98.68 40.87,100.41 Q12.2 | R115.2 41.01,98.54 | 41.01,98.54 40.87,98.68 | 41.01,98.54 40.98,98.54 40.87,98.42
  other vias: 34.54,77.93
LSRSTB  (via drill 0.1 pad 0.25 layers 15-16, 0.3 pad 0.51)
  Top 0.152: v34.98,79.88 35.2,79.65 R96.1 35.17,79.03
  GND1 0.076: v34.98,79.88 35.63,79.23 35.63,77.82 35.45,77.64 35.45,77.42 U7.H9
  other vias: 35.74,77.13
M_SCL  (via drill 0.3 pad 0.51)
  Top 0.152: U11.24 62.46,57.38 60.43,57.38 59.77,58.04 59.77,59.41 57.68,61.49 55.6,61.49 52.43,64.66 50.44,64.66 47.88,67.23 47.88,73.79 46.46,75.21 46.46,80.09 v46.28,80.26 | R23.2 33.93,101.6 33.35,101.02 33.35,99.69 33.68,99.36 v34.39,99.36
  GND 0.152: U11.18 18.97,106.81 24.15,101.62 31.42,101.62 33.68,99.36 v34.39,99.36 35.16,99.36 36.32,98.2 36.32,97.33 v43.21,90.45
  Bottom 0.152: 33.91,94.11 33.91,94.36 | v46.28,80.26 46.46,80.44 46.46,83.39 43.05,86.79 43.05,90.04 43.21,90.19 v43.21,90.45 | R73.1 33.78,94.23 | 33.78,94.23 33.91,94.36 | 33.78,94.23 33.91,94.11 | 33.91,94.11 33.91,93.55 Q4.3 | 33.91,94.36 33.91,98.88 v34.39,99.36
M_SDA  (via drill 0.3 pad 0.51)
  Top 0.152: U11.23 57.84,61.8 55.7,61.8 52.53,64.97 50.55,64.97 48.18,67.34 48.18,74.09 46.76,75.51 46.76,80.54 46.46,80.85 46.46,81.25 v46.91,81.71 46.76,81.56 | R22.2 34.1,100.01 v33.91,99.82
  GND 0.152: U11.17 21.46,104.78 24.31,101.93 31.77,101.93 33.88,99.82 v33.91,99.82 | v33.91,99.82 35.18,99.82 36.61,98.4 36.61,97.5 43.1,91.01 43.51,91.01 v43.87,90.65 | v33.91,99.82
  Bottom 0.152: Q3.3 28.32,93.71 R71.1 29.02,94.41 29.02,94.42 29.46,94.87 30.15,94.87 30.45,94.57 31.53,94.57 31.83,94.87 33.25,94.87 33.6,95.22 33.6,99.52 v33.91,99.82 | v46.91,81.71 46.91,83.39 43.41,86.89 43.41,89.89 43.87,90.35 v43.87,90.65
MC2_CLK  (via drill 0.3 pad 0.51)
  Top 0.152: U6.1 26.4,92.95 v26.39,92.94
  GND 0.152: v26.39,92.94 24.51,91.06 24.51,89.48 24.41,89.38 24.21,89.38 24.11,89.48 24.11,90.5 24,90.6 23.8,90.6 23.7,90.5 23.7,88.98 23.6,88.88 23.39,88.88 23.29,88.98 23.29,90.02 23.19,90.12 22.99,90.12 22.88,90.02 22.88,88.42 22.78,88.32 22.58,88.32 22.48,88.42 22.48,89.66 22.38,89.76 22.17,89.76 22.07,89.66 22.07,88.52 21.89,88.34 v21.36,88.34
  Bottom 0.152: J4.5 20.92,87.9 v21.36,88.34
MC2_CMD  (via drill 0.3 pad 0.51)
  Top 0.152: v28.27,90.7 U6.5
  GND 0.152: v28.27,90.7 28.27,89.64 28.17,89.53 27.91,89.53 27.81,89.64 27.81,90.6 27.71,90.7 27.56,90.7 27.46,90.6 27.46,89.64 27.36,89.53 27.2,89.53 27.1,89.64 27.1,90.6 27,90.7 26.85,90.7 26.75,90.6 26.75,89.64 26.64,89.53 26.49,89.53 26.39,89.64 26.39,89.95 26.3,90.04 26.14,90.04 26.04,89.94 26.04,89.64 25.93,89.53 25.63,89.53 22.63,86.54 22.28,86.54 22.17,86.64 22.17,87.06 22.07,87.16 21.92,87.16 21.82,87.06 21.82,86.64 21.72,86.54 21.56,86.54 21.46,86.64 21.46,87.06 21.36,87.16 21.21,87.16 21.11,87.06 21.11,86.69 20.95,86.54 v20.57,86.54
  Bottom 0.203: J4.3 20.27,85.7 20.55,85.98 20.55,86.51 v20.57,86.54
MC2_DA0  (via drill 0.3 pad 0.51)
  Top 0.152: U6.9 31.67,91.45 32,91.79 v32,92.99
  GND 0.152: v21.01,89.08 20.85,88.92 20.85,88.07 21.07,87.85 23.54,87.85 26.85,91.16 29.95,91.16 31.77,92.99 v32,92.99
  Bottom 0.152: 19.57,90.07 J4.7
  Bottom 0.203: 19.57,90.07 20.22,90.07 21.01,89.28 v21.01,89.08
MCINS  (via drill 0.1 pad 0.25 layers 1-2, 0.1 pad 0.25 layers 15-16, 0.2 pad 0.41 layers 2-15, 0.3 pad 0.51)
  Top 0.152: v28.88,75.62 32.08,75.62 33.53,77.07 v36.29,77.07
  GND 0.152: v36.29,77.07 36.29,76.98 36.55,76.72 36.93,76.72 37.03,76.81 38.55,76.81 v38.63,76.73 | v28.88,75.62 28.83,75.56 28.02,75.56 23.34,80.24 21.87,80.24 v20.31,81.8
  GND1 0.076: U7.D7 | U7.D7 37.34,76.72 37.59,76.97 37.91,76.97 38.01,76.88 38.49,76.88 v38.63,76.73
  Bottom 0.152: J4.SA v20.31,81.8
  other vias: 37.34,76.33
MIC1_N
  Bottom 0.102: U7.N5 32.93,74.71 30.33,74.71 C55.1
MIC1_P
  Bottom 0.102: U7.P5 33.34,75.38 32.86,74.89 30.33,74.89 C58.1
MICBIAS0  (via drill 0.1 pad 0.25 layers 1-2, 0.1 pad 0.25 layers 15-16, 0.2 pad 0.41 layers 2-15)
  Top 0.152: R12.2 33.19,73.47 v33.2,73.48
  GND 0.152: v33.2,73.48 33.4,73.48 v33.6,73.69
  GND1 0.102: v33.6,73.69 33.9,73.98 33.9,74.59 34.44,75.13 U7.L4
  other vias: 34.54,75.13
MP3_OUTL  (via drill 0.3 pad 0.51)
  Top 0.305: L9.1 17.58,88.7
  Top 0.406: L9.1 17.36,88.32 v17.04,88.32 17.09,88.32
  Bottom 0.152: v17.04,88.32 17.04,87.96 15.88,86.79 15.88,74.76 19.18,71.45 27.74,71.45 29.72,73.43 32.85,73.43 U7.P1
MP3_OUTR  (via drill 0.3 pad 0.51)
  Top 0.305: L10.1 15.58,88.81
  Top 0.406: 15.58,88.81 15.58,88.76 v16,88.34
  Bottom 0.152: v16,88.34 16.03,88.32 16.03,87.96 14.86,86.79 14.86,74.86 18.98,70.74 27.99,70.74 30.38,73.13 33,73.13 33.74,73.87 U7.N1
N$1  (via drill 0.3 pad 0.51)
  Top 0.203: v59.11,83.67 59.65,83.67 R87.1
  Bottom 0.076: U1.F8 57.35,82.55 57.61,82.8 57.9,82.8 58.01,82.92 58.01,83.21 58.09,83.29 58.45,83.29
  Bottom 0.152: 58.45,83.29 58.55,83.29 58.93,83.67 v59.11,83.67
N$2
  Bottom 0.132: C27.1 75.5,102.16 R79.1 C85.1
N$3  (via drill 0.3 pad 0.51)
  Top 0.152: v59.21,84.38 59.58,84.38 R92.1
  Bottom 0.076: U1.G9 57.76,83.18 58.01,83.44 58.01,83.72 58.09,83.8 58.45,83.8
  Bottom 0.152: 58.45,83.8 58.55,83.8 59.13,84.38 v59.21,84.38
N$4
  Bottom 0.152: U18.10 25.67,98.06 26.39,98.78 27.15,99.54 32.42,99.54 R69.2
N$5
  Bottom 0.406: J4.1 21.29,83.5 R74.2
N$6
  Bottom 0.132: U9.1 C24.1
N$7
  Bottom 0.152: U1.A1 50.9,80.05 C6.1
N$8
  Bottom 0.203: 56.76,77.11 C20.2
  Bottom 0.254: U1.A7 56.76,79.84 57.18,79.43 57.18,77.25 C20.2
N$9  (via drill 0.3 pad 0.51)
  Top 0.254: R4.2 55.91,77.51 v56.13,77.28
  Bottom 0.203: C15.1 55.5,77.09 | 56.12,77.29 v56.13,77.28
  Bottom 0.254: U1.A6 56.26,79.73 56.72,79.27 56.72,77.86 v56.13,77.28 55.94,77.09 55.5,77.09
N$10
  Bottom 0.132: C85.2 GPS.D
  Bottom 0.254: C85.2 77.22,101.23 77.22,100.58 76.33,99.69 72.01,99.69 71.75,99.44 L20.1
N$11
  Top 0.152: R28.1 34.62,98.17 35.38,98.93 36.24,98.93 J1.1
N$12
  Bottom 0.152: U1.A3 54.38,79.68 54.28,79.68 53.37,78.77 53.37,78.28
  Bottom 0.406: 53.37,78.28 53.37,77.95 52.6,77.19 52.6,76.66 L6.2
N$13
  Bottom 0.132: U13.3 L5.2
N$14
  Bottom 0.132: C25.1 U9.4
N$15
  Top 0.152: 45.77,98.93 J11.1 44.25,99.01 41.78,96.54 41.38,96.54 37.52,100.41 36.13,100.41 R23.1
N$16
  Bottom 0.152: U2.5 58.07,97.37 arc45 58.44,97.53 59.18,98.27 59.18,98.59 C43.1
N$17
  Top 0.406: R7.2 8.97,86.49 8.71,86.74 8.73,86.75 C148.+
N$18
  Bottom 0.152: U13.5 63.55,100.2 63.73,100.03 64.91,100.03 R41.1
N$19
  cutout GND: 56.87,81.91 57.63,81.91 57.63,81.13 57.02,81.13 57.02,80.14 56.87,80.14
  cutout GND1: 56.87,82.32 59.31,82.32 59.31,82.22 56.97,82.22 56.97,78.97 56.87,78.97
  cutout GND: 50.42,80.95 51.23,80.95 51.23,80.85 51.23,80.34 51.23,80.19 50.42,80.19
  cutout GND1: 50.42,80.95 51.23,80.95 51.23,80.85 51.23,80.34 51.23,80.19 50.42,80.19
  cutout GND1: 53.16,76.66 53.98,76.66 53.98,76.56 53.97,76.05 53.97,75.9 53.16,75.9
  cutout GND: 53.16,76.66 53.98,76.66 53.98,76.56 53.97,76.05 53.97,75.9 53.16,75.9
N$20  (via drill 0.3 pad 0.51)
  Top 0.152: v29.97,82.93 29.97,82.17 29.72,81.91 SW1.B
  Bottom 0.152: R19.2 29.34,82.68 29.59,82.93 v29.97,82.93
N$21
  cutout GND1 (isolate 0.254): 60.83,99.44 66.42,99.44 66.42,94.11 60.83,94.11
N$22
  pour Top (isolate 0.254, rank 2, no thermals): 28.45,61.34 22.48,61.34 arc-90 21.84,61.98 21.84,66.07 arc-90 22.48,66.71 23.62,66.71 arc-90 24.26,66.07 24.26,65.53 arc90 24.89,64.9 28.32,64.9 28.45,64.9 arc-90 29.08,64.26 29.08,61.98 arc-90
N$23
  Top 0.152: J1.2 34.07,97.01 R27.1
N$24
  Top 0.305: L9.2 18.63,89.57 C51.1
N$25
  Top 0.305: L10.2 14.69,89.78 C52.1
N$26
  Top 0.305: R10.1 17.79,92.19 C51.2
N$27
  Top 0.305: R11.1 14.69,92.44 C52.2
N$28  (via drill 0.3 pad 0.51)
  Top 0.305: R12.1 32.27,73.13 32.28,73.13 31.42,73.99 28.93,73.99 v28.52,74.4
  Bottom 0.203: C55.2
  Bottom 0.305: 28.98,74.26 C55.2 | R13.2 26.14,74.36 C57.1 | R13.2 C59.2 28.11,74.4 v28.52,74.4 28.92,74.4 C55.2 | 28.96,74.36 C55.2 | C60.1 27.05,72.92 arc-45 27.03,72.98 R13.2
N$29  (via drill 0.3 pad 0.51)
  Top 0.076: C96.1 31.7,77.42 v31.72,77.44
  Bottom 0.076: 33.72,77.51 U7.N10 33.72,77.5 32.74,77.5 32.61,77.5 31.78,77.5 v31.72,77.44
N$30
  Top 0.152: 29.03,96.44 29.21,96.27 RX.+ 29.21,97.41 Q6.3
N$31  (via drill 0.1 pad 0.25 layers 1-2, 0.1 pad 0.25 layers 15-16, 0.2 pad 0.41 layers 2-15, 0.3 pad 0.51)
  Top 0.152: v34.98,80.82 34.98,80.95 34.67,81.25 32.61,81.25 32.05,81.81 30.1,81.81 29.57,81.28 26.92,81.28 26.16,82.04 25.4,82.04 v25.02,82.42
  GND 0.102: 35.64,79.88 v35.64,79.73 | 35.64,79.88 35.59,79.88 | 35.64,79.88 35.64,79.94 34.98,80.6 v34.98,80.82
  GND 0.152: v25.02,82.42 23.19,84.25 12.73,84.25 11.56,85.42 v11.28,85.42
  GND1 0.076: U7.H10 35.78,77.57 35.78,79.59 v35.64,79.73
  Bottom 0.076: U7.H10 35.74,77.55
  Bottom 0.152: 11.76,84.94 v11.28,85.42 12.62,84.07 12.62,74.35 17.09,69.88 17.09,65.56 16.4,64.86 16.4,61.04 16.94,60.5 18.2,60.5 R47.1 | U7.H10
  other vias: 35.73,77.53
N$32
  Bottom 0.61: D15.- 32.87,58.83 U11.30
N$33
  Bottom 0.132: R21.1 79.93,83.31 | 79.93,83.31 WI-FI/BT.D | C84.1 79.81,83.44 79.93,83.31
N$34
  Top 0.152: U12.6 14.92,76.22 15.09,76.05 15.09,73.77 R33.2
N$35
  Top 0.406: U20.1 17,68.41 R30.2
N$36
  Top 0.203: C157.2 14.99,68.2 15.49,68.2 15.88,68.58 R30.1
N$38
  Top 0.305: U20.2 16.88,67.76 16.88,67.75 R91.2 R62.2
N$39
  Top 0.152: R76.1 29.16,100.28 Q6.2
N$40
  Top 0.152: J11.2 45.83,97.03 42.82,97.03 42.04,96.24 41.22,96.24 37.36,100.1 35.45,100.1 R22.1
  Top 0.203: 45.84,97 J11.2
N$41
  Bottom 0.406: J4.2 21.25,84.6 R2.2
N$42
  Bottom 0.132: C137.1 77.43,78.31 arc90 78.92,79.8 R21.2 78.92,83.33 C115.1
N$43
  Top 0.152: R77.1 26.19,100.48 Q7.2
N$44
  Top 0.152: 14.24,76.89 U12.5
  Top 0.203: 14.24,76.89 14.24,78 R48.1
N$45
  Top 0.203: R48.2 C105.2
N$46
  Top 0.152: U12.8 13.11,74.92 R50.1
N$47
  Top 0.152: U12.7 13.17,75.57 C77.1
N$48
  Top 0.152: C78.1 13.04,73.69 R51.2
N$49
  Bottom 0.152: 36.91,70.95 C104.1
  Bottom 0.203: 36.91,70.95 36.97,70.95 37.01,70.99 37.01,72.62 37.34,72.95 U7.D1 37.34,73.91
N$50
  Top 0.152: 19.99,78.13 20.95,77.16 20.7,77.16 20.64,77.1
  Top 0.203: U12.3 15.8,76.22 15.24,76.78 C105.1
  Top 0.406: U12.3 19.76,76.22 20.64,77.1 21.34,77.8
  pour Top (isolate 0.254, no thermals): 16.26,76.02 22.99,76.02 arc90 23.37,76.4 23.37,78.87 arc90 22.99,79.25 18.67,79.25 arc90 18.29,78.87 18.29,77.43 arc-90 17.39,76.53 16.26,76.53
N$51
  Top 0.152: C100.1 16.1,74.73 16.38,75.01 16.73,75.01 U12.1
N$52
  Top 0.152: R35.1 R50.2 R51.1 12.08,73.39 12.07,73.38 12.07,72.77 R34.1
N$55  (via drill 0.3 pad 0.51)
  Top 0.305: J16.1 v2.42,99.13 v2.41,99.14 | L21.2 16.64,102.72 v16.59,102.77
  GND 0.203: v2.41,99.14 2.41,99.78 5.4,102.77 v16.59,102.77
N$56
  Top 0.305: R78.1 13.4,57.97 PWR.+
N$57  (via drill 0.3 pad 0.51)
  Top 0.203: v24.77,58.67 RST.+
  Bottom 0.203: v24.77,58.67 23.81,59.63 R36.1
N$58
  Bottom 0.203: U2.47 56.54,101.01 R52.2
N$59
  Top 0.254: U20.8 C158.1
N$60
  Bottom 0.152: J4.8 20.4,91.2 22.12,89.48 22.12,87.72 R72.2
N$61
  Bottom 0.203: U2.33 51.17,97.77 50.57,98.37 R26.2
N$62
  Bottom 0.132: L4.1 L14.1 L12.2 C113.1
N$63
  Bottom 0.132: L4.2 C112.1
N$64
  Bottom 0.152: C43.2 63.84,98.6 arc-90 64.26,98.18 64.26,97.51 X2.3
N$65
  Bottom 0.132: L5.1 C25.2
N$66
  Bottom 0.132: C111.2 L15.2
N$67
  Bottom 0.132: C118.1 U13.6
N$68
  Bottom 0.132: C68.1 60.07,101.56 60.07,101.47 60.14,101.41 C67.1 C118.2
N$69
  Bottom 0.203: U2.32 50.44,97.37 R31.2
N$70
  Bottom 0.152: U2.40 53.74,100.3 R80.2
N$71
  Top 0.305: J16.6 3.42,106.3 | 3.42,106.3 3.42,106.86 R40.2 | R53.1 5.52,106.87 4.95,106.3 3.94,106.3 3.56,106.3 | 3.56,106.3 3.42,106.3 | 3.56,106.3 3.43,106.43 | 3.56,106.3 3.43,106.17
N$72
  Bottom 0.132: C124.1 79.83,65.55 R54.1 GSM.D
N$73
  Bottom 0.132: C83.1 R1.2 65.89,69.06 arc-45 68.01,68.18 69.73,66.47 arc45 71.98,65.53 R54.2 78.94,65.55 C125.1
N$74
  Bottom 0.152: U14.31 54.06,65.5 C130.1 R55.1
N$75
  Bottom 0.152: 54.55,63.07 R56.1 54.08,63.08 | 54.08,63.08 R57.1 | 54.08,63.08 54.08,64.45 C131.1 54.56,65.03 U14.30
N$76
  Bottom 0.132: U14.16 57.83,71.61 arc45 57.74,71.82 57.42,72.15 arc45 56.83,72.39 56.3,72.39 arc-45 55.58,72.69 55.52,72.75 arc45 55.22,72.87 50.17,72.87 arc45 49.9,72.76 47.46,70.32 arc-45 47,70.13 43.04,70.13 C132.1 42.06,70.14 L17.1
N$77
  Bottom 0.132: U14.15 57.33,71.54 arc90 56.92,71.96 50.53,71.96 arc45 50.26,71.84 47.58,69.17 arc-45 47.08,68.96 42.99,68.96 C133.1 42.96,68.96 L19.1
N$78
  Bottom 0.203: Q14.1 3.3,64.13 3.3,62.86 4.25,61.91 U8.3 4.19,61.53 4.19,61.47 4.57,61.09 Q1.3
N$80
  Bottom 0.132: U14.4 53.16,68.44 arc-45 53.02,68.49 52.77,68.75 arc45 52.62,68.81 L1.1
N$81
  Bottom 0.132: U14.3 53.16,67.94 arc45 52.98,67.86 52.76,67.64 arc-45 52.63,67.59 L16.1
N$82
  Bottom 0.203: U14.7 52.19,69.94 C136.1
N$83
  Bottom 0.152: U14.29 55.06,65.55 C129.1 55.66,64.99 56.16,64.49 56.16,63.61 R60.1
N$84
  Top 0.406: C107.+ 23.88,86.83 23.88,85.98 23.56,85.66 C93.1 22.61,85.09 22.48,85.22 22.48,85.15 R8.2
N$85
  Bottom 0.132: U15.1 69.12,78.81 C138.2
N$86
  Top 0.152: TX.+ 26.04,97.41 Q7.3
N$88
  Bottom 0.132: C138.1 U16.6
N$89
  Bottom 0.132: U16.4 71.08,76.91 C145.1
N$90
  Bottom 0.132: U16.2 C137.2
N$91
  Top 0.152: L.+ 22.17,96.19 21.72,96.65 21.72,97.54 21.97,97.79 21.97,101.37 22.16,101.55 22.72,101.55 R49.1
N$94
  Top 0.152: L.- 24.38,96.58 24.38,97.41 Q2.3
N$95  (via drill 0.3 pad 0.51)
  Top 0.203: SW1.A 28.07,86.49
  Top 0.406: 28.07,86.49 27.94,86.49 v27.43,87
  Bottom 0.406: v27.43,87 27.94,87 28.7,86.23 28.7,85.28 R20.2
N$96
  cutout GND1: 41.28,75.11 45.24,75.11 45.24,71.96 41.28,71.96
  cutout Bottom: 41.28,75.11 45.24,75.11 45.24,71.96 41.28,71.96
N$104  (via drill 0.1 pad 0.25 layers 1-2, 0.3 pad 0.51)
  Top 0.152: R105.2 34.18,71.13 v33.66,70.61
  Top 0.203: SW2.COM 3.99,71.4 3.99,71.61 | 3.99,71.61 v3.91,71.68 | 3.99,71.61 SW2.A
  GND 0.152: v33.66,70.61 29.72,70.61 28.83,71.5 13.72,71.5 9.65,75.56 5.33,75.56 3.94,74.17 3.94,74.04 3.91,74.02 v3.91,71.68
N$105
  Bottom 0.132: C24.2 R79.2 74.61,102.18 C117.1
N$106  (via drill 0.3 pad 0.51)
  Top 0.305: J16.4 8.52,104.13 8.87,103.78 v9.27,103.78 | L22.2 18.82,102.13 18.11,102.84 v17.91,102.84
  GND 0.152: v9.27,103.78 9.3,103.78 9.42,103.66 17.09,103.66 v17.91,102.84
  GND 0.305: v17.91,102.84 17.91,102.89
N$107  (via drill 0.3 pad 0.51)
  Top 0.203: v13.95,101.83 14.3,101.83 L23.2
  Top 0.305: 14.58,102.11 L23.2 | 14.38,102.36 L23.2 | J16.7 v6.32,101.78 v6.33,101.78 | 14.55,102.08 L23.2 | v8.26,99.34 8.26,97.68 J16.3
  GND 0.203: v6.33,101.78 6.33,101.27 v8.26,99.34 11.46,99.34 v13.95,101.83
N$108
  Top 0.152: R106.1 Q6.1
N$109
  Top 0.152: R107.1 Q7.1
N$110
  Top 0.152: Q2.1 24.41,100.31 R108.2 R29.2
N$111
  Bottom 0.203: U2.31 50.71,96.97 R109.2
N$112
  Bottom 0.152: U2.41 54.14,100.79 R110.2
PALDO_3V3  (via drill 0.3 pad 0.51)
  Top 0.203: 56.03,79.05 56.01,79.07
  Top 0.406: v58.57,78.94 58.57,78.51 58.6,78.49
  Top 0.61: v55.75,81.64 56.01,81.38 56.01,79.07 v56.01,78.92 56.01,78.55 56.06,78.5 | 57.52,78.25 C152.2 | R4.1 56.06,78.5 | 56.06,78.5 56.11,78.5 | 56.11,78.5 56.76,78.5 57.02,78.23 57.35,78.23 C152.2 | C152.2 57.71,78.16 58.04,78.49 58.6,78.49 58.91,78.49 C18.2 | 56.13,78.52 56.11,78.5
  Bottom 0.076: U1.E5 55.77,82.05
  Bottom 0.152: U1.A9 57.77,80.05 | U1.A5 55.76,79.69 56.01,79.44 v56.01,78.92 | U1.A9 57.76,80.01 | U1.A9 58.45,79.36 arc-45 58.52,79.18 58.52,78.99 v58.57,78.94
  Bottom 0.203: U1.E5 v55.76,81.64 v55.75,81.64
  Bottom 0.406: U15.2 68.9,78.16 C140.1 C139.1
  Bottom 0.61: v58.57,78.94 58.57,77.76 60.44,75.89 67.97,75.89 C139.1
PB1/D9/PWM1  (via drill 0.3 pad 0.51)
  Top 0.152: v28.93,103.81 28.93,103.96 29.54,104.57 36.37,104.57 38.61,106.81 U11.10
  Bottom 0.152: v28.93,103.81 U18.16
PD0/RX  (via drill 0.3 pad 0.51)
  Top 0.152: U11.1 61.6,104.78 39.5,104.78 38.08,103.35 34.67,103.35 | R28.2 33.01,98.2 33.01,102.45 33.91,103.35 34.37,103.35 | 34.37,103.35 34.67,103.35 | v34.52,102.89 34.52,103.2 | 34.52,103.2 34.67,103.35 | 34.52,103.2 34.37,103.35
  Bottom 0.152: R111.1 34.51,102.88 v34.52,102.89 34.52,103.2 34.87,103.56 Q9.3
PD1/TX  (via drill 0.3 pad 0.51)
  Top 0.152: R27.2 32.28,97.9 v32.28,100.05 32.28,102.23 33.72,103.66 37.92,103.66 39.35,105.08 59.36,105.08 U11.2
  Bottom 0.152: 35.26,99.39 R83.1 35.26,100.28 | 37.29,100.08 Q8.3 37.11,100.35 35.58,100.35 35.33,100.35 | 35.26,100.28 35.33,100.35 | v32.28,100.05 32.28,100.24 32.76,100.71 34.98,100.71 35.26,100.43 | 35.26,100.28 35.26,100.43 | 35.33,100.35 35.26,100.43
PD2/INT0  (via drill 0.3 pad 0.51)
  Top 0.152: v41.43,97.77 43.31,99.64 43.31,103.76 43.71,104.16 44.32,104.16 v44.88,103.61
  Bottom 0.152: Q11.3 38.99,93.47 38.99,96.31 40.08,97.4 40.76,97.4 41.12,97.77 v41.43,97.77 | 44.88,103.35 44.88,103.45 55.19,103.45 U11.3 | 44.89,103.45 v44.89,103.6 v44.88,103.61
  Bottom 0.203: 44.89,103.01 R116.1 44.88,103.45 v44.88,103.61
PD3/INT1/PWM0  (via drill 0.3 pad 0.51)
  Top 0.152: v29.59,103.76 29.59,104.01 29.84,104.27 37.31,104.27 37.59,104.27 38.99,105.66 42.98,105.66 45.39,108.08 54.74,108.08 U11.4
  Bottom 0.152: U18.17 29.57,103.74 v29.59,103.76
PD4  (via drill 0.3 pad 0.51)
  Top 0.152: v40.41,98.22 41.07,98.22 43,100.16 43,104.11 43.36,104.47 53.06,104.47 v53.52,104.01
  Bottom 0.152: R113.1 36.72,95.95 Q10.3 38.44,96.57 39.86,98 40.19,98 v40.41,98.22 | v53.52,104.01 53.52,106.76 U11.5
PD5/PWM  (via drill 0.3 pad 0.51)
  Top 0.152: v31.57,103.45 32.08,103.96 37.72,103.96 39.14,105.38 49.51,105.38 U11.6
  Bottom 0.152: U18.20 31.52,103.41 v31.57,103.45
PD6/PWM
  Bottom 0.152: U18.18 30.22,103.63 30.71,104.11 36.35,104.11 37.92,105.69 37.92,107.62 38.43,108.13 47.07,108.13 U11.7
PD7  (via drill 0.3 pad 0.51)
  Top 0.152: v41.53,97.1 43.87,99.44 v43.87,103.61
  Bottom 0.152: v41.53,97.1 41.17,97.1 Q13.3
  Bottom 0.203: U11.8 43.87,104.83 v43.87,103.61 R119.1
PWRKEY  (via drill 0.1 pad 0.25 layers 1-2, 0.1 pad 0.25 layers 15-16, 0.2 pad 0.41 layers 2-15)
  Top 0.102: R105.1 35.87,73.1 v35.89,73.13
  GND 0.102: v36.55,74.24 36.45,74.24 36.25,74.04 36.25,73.48 v35.89,73.13
  GND1 0.076: v36.22,74.85 36.25,74.85 36.55,74.55 v36.55,74.24
  Bottom 0.102: v36.22,74.85 36.22,75.05 U7.G4
RESET  (via drill 0.3 pad 0.51)
  Top 0.152: RST.- 25.53,57.63 v25.5,57.66 | v16.84,59.59 17.63,59.59 RESET.1
  Top 0.203: 17.5,59.41 RESET.1 | 17.65,59.97 17.4,59.97
  Top 0.406: RESET.1 17.65,59.97
  Bottom 0.152: JTAG.5 14.96,103.15 14.91,103.15 14.61,102.84 14.61,95.83 12.01,93.24 12.01,86.89 10.8,85.68 10.8,85.21 12.32,83.69 12.32,74.19 16.76,69.75 16.76,65.66 16.07,64.97 16.07,60.36 v16.84,59.59 16.88,59.63 R47.2 | v25.5,57.66 25.48,57.63 25.07,57.63 23.6,59.11 20.75,59.11 20.24,59.61 R81.1 19.36,60.52 C81.1 19.11,60.52 18.22,59.63 R47.2 | 18.2,59.61 R47.2
  Bottom 0.406: v25.5,57.66 25.83,57.33 28.88,57.33 29.34,57.78 29.34,62.64 D15.+
RXHB_P
  Bottom 0.132: U7.B1 38.14,73.82 38.9,73.06 arc-45 38.99,72.85 38.99,71.34 arc45 39.17,70.9 L19.2
RXLB_P
  Bottom 0.132: L17.2 39.7,71.61 arc-45 39.6,71.86 39.6,72.74 arc45 39.51,72.96 U7.A1
SIM1_SCLK  (via drill 0.1 pad 0.25 layers 15-16, 0.2 pad 0.41 layers 2-15, 0.3 pad 0.51)
  GND 0.152: v33.5,75.26 33.5,75.62 33.3,75.82 32.74,75.82 32.32,75.4 31.18,75.4 28.57,78 28.57,83.13 28.27,83.44 28.27,87.5 27.46,88.32 26.19,88.32 23.05,85.18 13.02,85.18 9.88,88.32 9.88,94.11 v10.03,94.26
  GND1 0.076: U7.K7 34.94,76.29 34.82,76.17 34.82,76.01 34.08,75.26 v33.5,75.26
  Bottom 0.152: C62.1 10.21,97.09 J4.C3 10.24,95.07 10.24,94.46 v10.03,94.26
  other vias: 34.94,76.33
SIM1_SIO  (via drill 0.1 pad 0.25 layers 15-16, 0.2 pad 0.41 layers 2-15, 0.3 pad 0.51)
  GND 0.076: 32.72,76.73 32.94,76.73 33.64,76.04 34.1,76.04 34.31,76.25 34.31,76.99 v34.21,77.09
  GND 0.102: 32.72,76.73 32.64,76.73 31.97,76.06 31.48,76.06 30.86,76.68
  GND 0.152: 30.86,76.68 29.18,78.36 29.18,83.44 28.88,83.74 28.88,87.86 27.81,88.92 25.88,88.92 22.73,85.77 13.34,85.77 10.49,88.62 10.49,93.27 v10.67,93.45
  GND1 0.102: U7.L9 34.25,77.13 v34.21,77.09
  Bottom 0.152: C64.1 J4.C7 11.48,94.26 v10.67,93.45
  other vias: 34.54,77.13
SIM1_SRST  (via drill 0.1 pad 0.25 layers 15-16, 0.2 pad 0.41 layers 2-15, 0.3 pad 0.51)
  GND 0.152: v32.83,76.35 32.24,75.76 31.32,75.76 28.88,78.21 28.88,83.29 28.57,83.59 28.57,87.71 27.66,88.62 26.04,88.62 22.89,85.47 13.18,85.47 10.85,87.8 | 10.79,87.85 10.85,87.8 | v7.67,94.39 8.1,94.82 10.24,94.82 10.54,94.51 10.54,94 10.19,93.65 10.19,88.47 10.85,87.8
  GND1 0.076: U7.K8 34.87,76.73 34.75,76.61 34.04,76.61 33.61,76.17 33.01,76.17 v32.83,76.35
  Bottom 0.152: 7.64,95.08 J4.C2 | J4.C2 7.67,97.07 C61.1 | v7.67,94.39 J4.C2
  other vias: 34.94,76.73
SMPSLDO_1V6  (via drill 0.3 pad 0.51)
  Top 0.152: 54.28,80.85 v54.28,80.77 54.28,80.64
  Top 0.203: C16.2 59.66,82.73 59.31,82.37 v58.83,82.37 | C19.2 v57.81,79.2 | C17.2 59.18,81.84 v59.11,81.76
  Top 0.305: C13.2 54.03,81.03 v54.28,80.77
